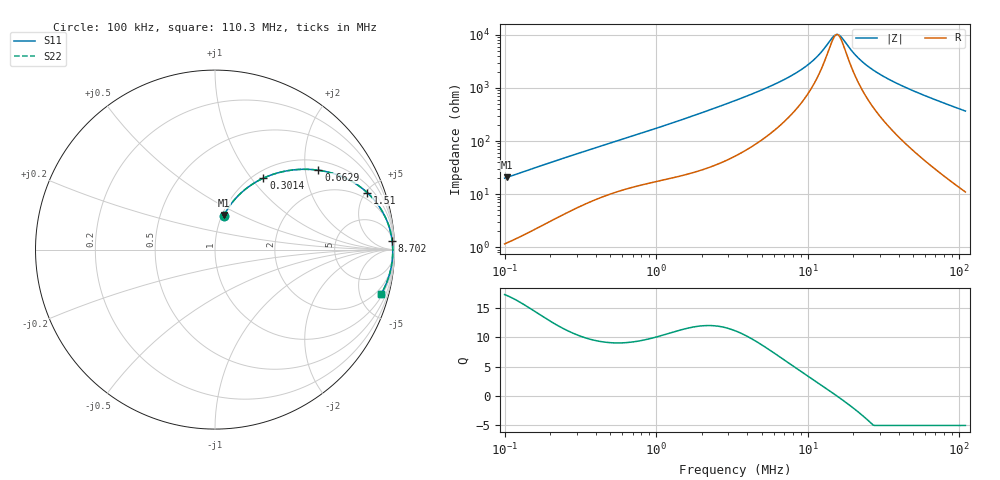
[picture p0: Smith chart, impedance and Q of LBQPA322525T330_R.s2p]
! LBQPA322525T330_R  S-PARAMETER MODEL  ( General Type )
! Model Generated by TAIYO YUDEN Corporation (http://www.ty-top.com)
! Version 1.0
! TAIYO YUDEN Control No. 191025NI43SB-FBB
! Copyright(c) 2019 TAIYO YUDEN CO.,LTD. All Rights Reserved.
! Product Description (link to TY-COMPAS)
! https://ds.yuden.co.jp/TYCOMPAS/or/detail?pn=LBQPA322525T330KR&u=M
! Products Name : Inductors
! Characteristics :
!  Inductance : 33 uH , SRF(min) : 13 MHz , DC Resistance(max) : 0.533 Ohm
!  Rated Current : Saturation :500 mA , Temp Rise : 400 mA (20 degC)
!  Case Size : 3.2 x 2.5 / 0.126 x 0.098 [mm/inch] , Thickness : 2.5 / 0.098 [mm/inch]
!  (Conditions: Temperature = 25 degC , DC Bias Current/Voltage = 0A / 0V)
! External Node Assignments :
!  1  o---GGG---o  2
! GND o---------o GND
! Frequency Range : 0.1MHz  -  110.285862MHz  [ 402 STEP ]
# MHz S RI R 50
! Freq[MHz].  S11 Real  S11 Imag  S21 Real  S21 Imag  S12 Real  S12 Imag  S22 Real  S22 Imag
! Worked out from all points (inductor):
!   401 points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, 100 kHz to 110.3 MHz, reference 50 ohm
!   read as one part in series: L = 31.6 uH near 103.6 kHz
!   highest Q = 17.1 at 103.6 kHz (marker M1), where L = 31.7 uH
!   self-resonance near 15.51 MHz
!   S11 on the Smith chart (normalised r, x): 100 kHz: 1.02, +0.40; 301.4 kHz: 1.11, +1.15; 662.9 kHz: 1.26, +2.36; 1.51 MHz: 1.45, +5.13; 8.702 MHz: 10, +40; 110.3 MHz: 1.22, -7.33
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0.1  0.0485 0.1877  0.9515 -0.1877  0.9515 -0.1877  0.0485 0.1877
0.103565  0.0515 0.1936  0.9485 -0.1936  0.9485 -0.1936  0.0515 0.1936
0.18139  0.1308 0.3018  0.8692 -0.3018  0.8692 -0.3018  0.1308 0.3018
0.301437  0.2696 0.3981  0.7304 -0.3981  0.7304 -0.3981  0.2696 0.3981
0.323312  0.2938 0.4085  0.7062 -0.4085  0.7062 -0.4085  0.2938 0.4085
0.662949  0.5759 0.4423  0.4241 -0.4423  0.4241 -0.4423  0.5759 0.4423
1.045308  0.7452 0.3892  0.2548 -0.3892  0.2548 -0.3892  0.7452 0.3892
1.509998  0.8483 0.3173  0.1517 -0.3173  0.1517 -0.3173  0.8483 0.3173
3.320932  0.957 0.1627  0.043 -0.1627  0.043 -0.1627  0.957 0.1627
5.816497  0.9807 0.0865  0.0193 -0.0865  0.0193 -0.0865  0.9807 0.0865
8.701746  0.9872 0.0468  0.0128 -0.0468  0.0128 -0.0468  0.9872 0.0468
10.73698  0.9889 0.0292  0.0111 -0.0292  0.0111 -0.0292  0.9889 0.0292
12.35186  0.9896 0.0181  0.0104 -0.0181  0.0104 -0.0181  0.9896 0.0181
14.71619  0.9901 0.00465  0.00985 -0.00465  0.00985 -0.00465  0.9901 0.00465
15.78413  0.9903 -0.000672  0.00974 0.000672  0.00974 0.000672  0.9903 -0.000672
16.63564  0.9903 -0.00467  0.0097 0.00467  0.0097 0.00467  0.9903 -0.00467
20.17013  0.9902 -0.0196  0.00983 0.0196  0.00983 0.0196  0.9902 -0.0196
23.2038  0.9898 -0.0309  0.0102 0.0309  0.0102 0.0309  0.9898 -0.0309
27.64535  0.9888 -0.0459  0.0112 0.0459  0.0112 0.0459  0.9888 -0.0459
34.71395  0.9866 -0.0676  0.0134 0.0676  0.0134 0.0676  0.9866 -0.0676
57.68817  0.9745 -0.1297  0.0255 0.1297  0.0255 0.1297  0.9745 -0.1297
110.2859  0.9244 -0.2498  0.0756 0.2498  0.0756 0.2498  0.9244 -0.2498
